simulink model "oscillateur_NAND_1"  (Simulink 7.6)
settings: Solver=ode15s  StartTime=0.0  StopTime=0.01  RelTol=1e-3
StopFcn:
  | close all, clc
  | load signaux.mat
  | plot(x(1,:),x(2,:))
  | grid
  | title('Oscillateur à portes NAND, T=2RC ln3 ou 2.2 RC???')
  | 
  | xlabel('temps')
  | axis([0 0.01 -0.1 1.1])
libraries: elec_lib x5, fl_lib x4, nesl_utility x3

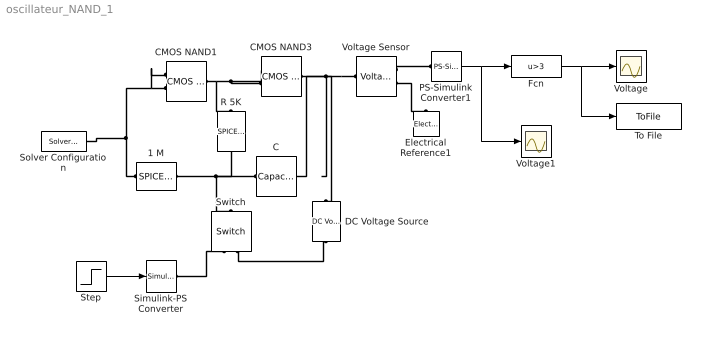
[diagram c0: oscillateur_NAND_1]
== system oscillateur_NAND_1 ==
  1 M : elec_lib/Additional Components/SPICE-Compatible Components/Passive Devices/SPICE Resistor  DialogController=NetworkEngine.DynNeDlgSource  SystemSampleTime=-1  SCALE=1  R_param=1  R=1e3 kOhm  RSH=0 Ohm  LENGTH=1e-06 m  WIDTH=1e-06 m  NARROW=0 m  T_param=1  TC1=0 1/K  TC2=0 1/K^2  TOFFSET=0 K  TFIXED=300.15 K  TMEAS=300.15 K  LocalVarLogging=[]
  C : fl_lib/Electrical/Electrical Elements/Capacitor  DialogController=NetworkEngine.DynNeDlgSource  SystemSampleTime=-1  c=100e-9 F  v0=0 V  r=1e-6 Ohm  g=0 1/Ohm  i_Log=off  v_Log=off  vc_Log=off  LocalVarNames=|current|voltage|power  LocalVarDescs=|Capacitor current (A)|Voltage across capacitor (V)|Power (W)  LocalVarLogging=[0 0 0]
  CMOS NAND1 : elec_lib/Integrated Circuits/Logic/CMOS NAND  DialogController=NetworkEngine.DynNeDlgSource  SystemSampleTime=-1  V_IL=2 V  V_IH=3 V  C_IN=5 pF  output_type=1  V_OL=0 V  V_OH=5 V  V_CC=5 V  V_meas=5 V  R_OUT=450 Ohm  R_OH=[ 25 250 ] Ohm  I_OH=63 mA  R_OL=[ 30 800 ] Ohm  I_OL=-45 mA  Delay=1.2e-07 s  Ron=5 Ohm  Vf=0.6 V  output_state=1  LocalVarLogging=[]
  CMOS NAND3 : elec_lib/Integrated Circuits/Logic/CMOS NAND  DialogController=NetworkEngine.DynNeDlgSource  SystemSampleTime=-1  V_IL=2 V  V_IH=3 V  C_IN=5 pF  output_type=1  V_OL=0 V  V_OH=5 V  V_CC=5 V  V_meas=5 V  R_OUT=450 Ohm  R_OH=[ 25 250 ] Ohm  I_OH=63 mA  R_OL=[ 30 800 ] Ohm  I_OL=-45 mA  Delay=1.2e-07 s  Ron=5 Ohm  Vf=0.6 V  output_state=1  LocalVarLogging=[]
  DC Voltage Source : elec_lib/Additional Components/SPICE-Compatible Components/Sources/DC Voltage Source  DialogController=NetworkEngine.DynNeDlgSource  SystemSampleTime=-1  DC=1 V  current_Log=off  voltage_Log=off  power_Log=off  LocalVarNames=|current|voltage|power  LocalVarDescs=|Current (A)|Voltage (V)|Power (W)  LocalVarLogging=[0 0 0]
  Electrical Reference1 : fl_lib/Electrical/Electrical Elements/Electrical Reference  DialogController=NetworkEngine.DynNeDlgSource  SystemSampleTime=-1  i_Log=off  LocalVarNames=|i  LocalVarDescs=|i  LocalVarLogging=[]
  Fcn : Fcn  Expr=u>3
  PS-Simulink Converter1 : nesl_utility/PS-Simulink Converter  DialogController=NetworkEngine.DynNeUtilDlgSource  SystemSampleTime=-1  PhysicalDomain=network_engine_domain  LeftPortType=input  RightPortType=output  SubClassName=ps_output  Unit=1  AffineConversion=off
  R 5K : elec_lib/Additional Components/SPICE-Compatible Components/Passive Devices/SPICE Resistor  DialogController=NetworkEngine.DynNeDlgSource  SystemSampleTime=-1  SCALE=1  R_param=1  R=5 kOhm  RSH=0 Ohm  LENGTH=1e-06 m  WIDTH=1e-06 m  NARROW=0 m  T_param=1  TC1=0 1/K  TC2=0 1/K^2  TOFFSET=0 K  TFIXED=300.15 K  TMEAS=300.15 K  LocalVarLogging=[]
  Simulink-PS Converter : nesl_utility/Simulink-PS Converter  DialogController=NetworkEngine.DynNeUtilDlgSource  SystemSampleTime=-1  PhysicalDomain=network_engine_domain  LeftPortType=input  RightPortType=output  SubClassName=ps_input  Unit=1  AffineConversion=off  InputFilterTimeConstant=.001  UdotUserProvided=0
  Solver Configuration : nesl_utility/Solver Configuration  DialogController=NetworkEngine.DynNeUtilDlgSource  SystemSampleTime=-1  PhysicalDomain=network_engine_domain  LeftPortType=input  RightPortType=generic  SubClassName=solver  Accelerate=off  Profile=off  ResidualTolerance=1e-9  MaxNonlinIter=12  MaxModeIter=2  DoFixedCost=off  UseLocalSampling=off  DoDC=off  LinearAlgebra=Sparse  LocalSolverSampleTime=.001  LocalSolverChoice=NE_BACKWARD_EULER_ADVANCER  UseLocalSolver=off
  Step : Step  Time=0.001  Before=1  After=0  SampleTime=0
  Switch : fl_lib/Electrical/Electrical Elements/Switch  DialogController=NetworkEngine.DynNeDlgSource  SystemSampleTime=-1  R_closed=0.01 Ohm  G_open=1e-08 1/Ohm  Threshold=0  i_Log=off  v_Log=off  LocalVarNames=|i|v  LocalVarDescs=|i|v  LocalVarLogging=[0 0]
  To File : ToFile  Filename=signaux  MatrixName=x
  Voltage : Scope
  Voltage Sensor : fl_lib/Electrical/Electrical Sensors/Voltage Sensor  DialogController=NetworkEngine.DynNeDlgSource  SystemSampleTime=-1  i1_Log=off  v1_Log=off  LocalVarNames=|i1|v1  LocalVarDescs=|i1|v1  LocalVarLogging=[0 0]
  Voltage1 : Scope
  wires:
  Step/1 -> Simulink-PS Converter/1
  PS-Simulink Converter1/1 -> Fcn/1, Voltage1/1
  Fcn/1 -> Voltage/1, To File/1
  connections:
  CMOS NAND1/RConn1 -- CMOS NAND3/LConn1 -- CMOS NAND3/LConn2 -- R 5K/LConn1
  Voltage Sensor/LConn1 -- C/LConn1 -- DC Voltage Source/LConn1 -- CMOS NAND3/RConn1
  1 M/LConn1 -- C/RConn1 -- R 5K/RConn1 -- Switch/LConn1
  CMOS NAND1/LConn2 -- 1 M/RConn1 -- Solver Configuration/RConn1 -- CMOS NAND1/LConn1
  Voltage Sensor/RConn2 -- Electrical Reference1/LConn1
  Voltage Sensor/RConn1 -- PS-Simulink Converter1/LConn1
  Switch/RConn2 -- DC Voltage Source/RConn1
  Simulink-PS Converter/RConn1 -- Switch/RConn1
